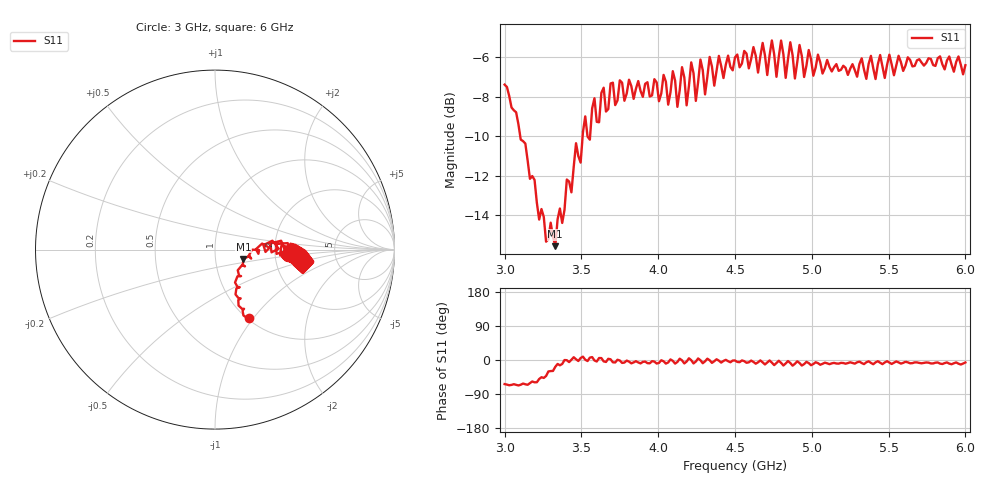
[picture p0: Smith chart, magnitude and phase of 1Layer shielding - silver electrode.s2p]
!  03/07/2025  15:14:19
! Ref Plane: 0.000 mm
# MHZ S MA R  50
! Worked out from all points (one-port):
!   201 points, 3 GHz to 6 GHz, reference 50 ohm
!   lowest |S11| = -15.6 dB at 3.33 GHz (marker M1), VSWR 1.40, Z = 68.4 - j7.26 ohm
!   |S11| at or under -10 dB: 3.102 GHz to 3.508 GHz (406.4 MHz wide, 12.3 % of centre); 3.539665 GHz to 3.556691 GHz (17.03 MHz wide, 0.48 % of centre)
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3000  0.4265 -63.6
3330  0.1669 -18.0
3375  0.191 -10.5
3525  0.3547 0.9
3750  0.4373 -1.3
4065  0.3797 -6.5
4095  0.4612 -2.2
4125  0.3749 -5.2
4155  0.4721 -0.9
4185  0.3782 -4.2
4215  0.4853 -0.5
4245  0.3881 -4.1
4275  0.4934 -0.6
4305  0.403 -3.5
4335  0.501 -0.7
4500  0.4997 -1.2
4695  0.5057 -11.8
4725  0.5053 -1.2
4755  0.5089 -13.5
4785  0.5014 -1.9
4815  0.5089 -14.5
4845  0.4944 -2.7
4875  0.5059 -14.9
4905  0.4849 -3.5
4935  0.504 -14.6
5250  0.4677 -6.1
5625  0.4999 -6.2
6000  0.4775 -6.5
